| (C) Copyright National Semiconductor Corporation 2008
| and Teraspeed Consulting Group LLC 2008
|   National Semiconductor Corporation
|   Data Conversion Products Group
|   IBIS Model of ADC08D1000QML
|   128 Pin Quad Gullwing Ceramic Package
| Teraspeed Modeling Services.
| http://www.teraspeed.com
[IBIS Ver]  3.2
[File Name] adc08d1000qml.ibs
[File Rev]  3.3
[Source]  Created by Teraspeed Consulting Group LLC
[Date]   06/02/2008
[Notes]   Quality Check of this IBIS model: Model Passes IBIS Check
   Model parses into ICX IS. Simulation done with Hyperlynx.
   1. MIN TYP MAX information is based on Temprature and
   Voltage characteristics only.
   2. Package data gained using TDA Systems Iconnect Software.
[Disclaimer]
   All rights reserved
|   National Semiconductor Corporation hereby grants
|the user of this IBIS model a non-exclusive, nontransferable
|license to use this IBIS model under the following terms.
|Before using this IBIS model, the user should read this
|license.  If the user does not accept these terms,  the
|IBIS model should be returned to National within 30 days.
|   The user is granted this license only to use the
|IBIS model and is not granted rights to sell, load, rent,
|lease or license the IBIS model in whole or in part, or in
|modified form to anyone other than user. User may modify
|the IBIS model to suit its specific applications but rights
|to derivative works and such modifications shall belong to
|National.
|   This IBIS model is provided on an "AS IS" basis and
|National makes absolutely no warranty with respect to the
|information contained herein.NATIONAL DISCLAIMS AND CUSTOMER
|WAIVES ALL WARRANTIES, EXPRESS OR IMPLIED, INCLUDING
|WARRANTIES OF MERCHANTABILITY OR FITNESS FOR A PARTICULAR
|PURPOSE. The entire risk as to quality and performance is
|with the Customer. ACCORDINGLY, IN NO EVENT SHALL THE
|COMPANY BE LIABLE FOR ANY DAMAGES, WHETHER IN CONTRACT OR
|TORT,INCLUDING ANY LOST PROFITS OR OTHER INCIDENTAL,
|CONSEQUENTIAL, EXEMPLARY, OR PUNITIVE DAMAGES ARISING OUT
|OF THE USE OR APPLICATION OF THE IBIS model provided in
|this package.Further, National reserves the right to make
|changes without notice to any product herein to improve
|reliability, function, or design. National does not convey
|any license under patent rights or any other intellectual
|property rights, including those of third parties.
|   National is not obligated to provide maintenance or support
|for the licensed IBIS model.
| Use: Teraspeed Consulting Group LLC ("Teraspeed") has
| licensed IBIS models to specific integrated circuit
| suppliers ("IC Vendors") for use and distribution as
| follows: Each IC Vendor may use IBIS Models, and distribute
| them to IC Vendor's custumers to use solely for developing
| printed circute board designs. Users of this model may
| modify the IBIS model to suit its specific applications but
| rights to derivative works and such modifications shell belong
| to Teraspeed. No other distribution of these materials is
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[Copyright]
| This file is the legal property of National Semiconductor and
| Teraspeed Copyright(c) 2008.
| All other rights are reserved.
[Component]   ADC08D1000QML
[Manufacturer] National Semiconductor
[Package]
| variable   typ   min   max
R_pkg  1.000E-02  1.000E-02  1.000E-02
L_pkg  9.028E-09  8.236E-09  1.114E-08
C_pkg  2.390E-12  2.180E-12  2.950E-12
[Pin] signal_name  model_name  R_pin  L_pin C_pin
1   GND   GND   1.000E-02   1.114E-08   2.950E-12
2   VA   POWER   1.000E-02   1.081E-08   2.862E-12
3   OUTV/SCLK   in_ctrl   1.000E-02   1.050E-08   2.779E-12
4   OUTEDGE/DDR/SDATA   in_3lvl   1.000E-02   1.020E-08   2.700E-12
5   VA   POWER   1.000E-02   9.918E-09   2.625E-12
6   GND   GND   1.000E-02   9.653E-09   2.555E-12
7   VCMO   term   1.000E-02   9.408E-09   2.490E-12
8   VA   POWER   1.000E-02   9.183E-09   2.431E-12
9   GND   GND   1.000E-02   8.979E-09   2.377E-12
10   VINI-   term   1.000E-02   8.798E-09   2.329E-12
11   VINI+   term   1.000E-02   8.640E-09   2.287E-12
12   GND   GND   1.000E-02   8.507E-09   2.252E-12
13   VA   POWER   1.000E-02   8.399E-09   2.223E-12
14   FSR/ECE   in_rst   1.000E-02   8.318E-09   2.202E-12
15   DCLK_RST   in_rst   1.000E-02   8.263E-09   2.187E-12
16   VA   POWER   1.000E-02   8.236E-09   2.180E-12
17   VA   POWER   1.000E-02   8.236E-09   2.180E-12
18   CLK+   in_lvds   1.000E-02   6.040E-09   1.890E-12
19   CLK-   in_lvds   1.000E-02   5.750E-09   1.900E-12
20   VA   POWER   1.000E-02   8.399E-09   2.223E-12
21   GND   GND   1.000E-02   8.507E-09   2.252E-12
22   VINQ+   term   1.000E-02   8.640E-09   2.287E-12
23   VINQ-   term   1.000E-02   8.798E-09   2.329E-12
24   GND   GND   1.000E-02   8.979E-09   2.377E-12
25   VA   POWER   1.000E-02   9.183E-09   2.431E-12
26   PD   in_pd   1.000E-02   9.408E-09   2.490E-12
27   GND   GND   1.000E-02   9.653E-09   2.555E-12
28   VA   POWER   1.000E-02   9.918E-09   2.625E-12
29   PDQ   in_ctrl   1.000E-02   1.020E-08   2.700E-12
30   CAL   in_rst   1.000E-02   1.050E-08   2.779E-12
31   VBG   term   1.000E-02   1.081E-08   2.862E-12
32   REXT   term   1.000E-02   1.114E-08   2.950E-12
33   VA   POWER   1.000E-02   1.114E-08   2.950E-12
34   TDIODE_P   term   1.000E-02   1.081E-08   2.862E-12
35   TDIODE_N   term   1.000E-02   1.050E-08   2.779E-12
36   DQD0+   out_lvds  1.000E-02   1.020E-08   2.700E-12
37   DQD0-   out_lvds  1.000E-02   9.918E-09   2.625E-12
38   DQD1+   out_lvds  1.000E-02   9.653E-09   2.555E-12
39   DQD1-   out_lvds  1.000E-02   9.408E-09   2.490E-12
40   VDR   POWER   1.000E-02   9.183E-09   2.431E-12
41   _ECE   in_ctrl   1.000E-02   8.979E-09   2.377E-12
42   DRGND   GND   1.000E-02   8.798E-09   2.329E-12
43   DQD2+   out_lvds  1.000E-02   8.640E-09   2.287E-12
44   DQD2-   out_lvds  1.000E-02   8.507E-09   2.252E-12
45   DQD3+   out_lvds  1.000E-02   8.399E-09   2.223E-12
46   DQD3-   out_lvds  1.000E-02   8.318E-09   2.202E-12
47   DQD4+   out_lvds  1.000E-02   8.263E-09   2.187E-12
48   DQD4-   out_lvds  1.000E-02   8.236E-09   2.180E-12
49   DQD5+   out_lvds  1.000E-02   8.236E-09   2.180E-12
50   DQD5-   out_lvds  1.000E-02   8.263E-09   2.187E-12
51   VDR   POWER   1.000E-02   8.318E-09   2.202E-12
52   DRST_SEL   in_ctrl   1.000E-02   8.399E-09   2.223E-12
53   DRGND   GND   1.000E-02   8.507E-09   2.252E-12
54   DQD6+   out_lvds  1.000E-02   8.640E-09   2.287E-12
55   DQD6-   out_lvds  1.000E-02   8.798E-09   2.329E-12
56   DQD7+   out_lvds  1.000E-02   8.979E-09   2.377E-12
57   DQD7-   out_lvds  1.000E-02   9.183E-09   2.431E-12
58   DQ0+   out_lvds  1.000E-02   9.408E-09   2.490E-12
59   DQ0-   out_lvds  1.000E-02   9.653E-09   2.555E-12
60   DQ1+   out_lvds  1.000E-02   9.918E-09   2.625E-12
61   DQ1-   out_lvds  1.000E-02   1.020E-08   2.700E-12
62   VDR   POWER   1.000E-02   1.050E-08   2.779E-12
63   NC   NC   1.000E-02   1.081E-08   2.862E-12
64   DRGND   GND   1.000E-02   1.114E-08   2.950E-12
65   DQ2+   out_lvds  1.000E-02   1.114E-08   2.950E-12
66   DQ2-   out_lvds  1.000E-02   1.081E-08   2.862E-12
67   DQ3+   out_lvds  1.000E-02   1.050E-08   2.779E-12
68   DQ3-   out_lvds  1.000E-02   1.020E-08   2.700E-12
69   DQ4+   out_lvds  1.000E-02   9.918E-09   2.625E-12
70   DQ4-   out_lvds  1.000E-02   9.653E-09   2.555E-12
71   DQ5+   out_lvds  1.000E-02   9.408E-09   2.490E-12
72   DQ5-   out_lvds  1.000E-02   9.183E-09   2.431E-12
73   VDR   POWER   1.000E-02   8.979E-09   2.377E-12
74   DRGND   GND   1.000E-02   8.798E-09   2.329E-12
75   DQ6+   out_lvds  1.000E-02   8.640E-09   2.287E-12
76   DQ6-   out_lvds  1.000E-02   8.507E-09   2.252E-12
77   DQ7+   out_lvds  1.000E-02   8.399E-09   2.223E-12
78   DQ7-   out_lvds  1.000E-02   8.318E-09   2.202E-12
79   OR+/DCLK2+   out_lvds  1.000E-02   8.263E-09   2.187E-12
80   OR-/DCLK2-   out_lvds  1.000E-02   8.236E-09   2.180E-12
81   DCLK-   out_lvds  1.000E-02   8.236E-09   2.180E-12
82   DCLK+   out_lvds  1.000E-02   8.263E-09   2.187E-12
83   DI7-   out_lvds  1.000E-02   8.318E-09   2.202E-12
84   DI7+   out_lvds  1.000E-02   8.399E-09   2.223E-12
85   DI6-   out_lvds  1.000E-02   8.507E-09   2.252E-12
86   DI6+   out_lvds  1.000E-02   8.640E-09   2.287E-12
87   DRGND   GND   1.000E-02   8.798E-09   2.329E-12
88   VDR   POWER   1.000E-02   8.979E-09   2.377E-12
89   DI5-   out_lvds  1.000E-02   9.183E-09   2.431E-12
90   DI5+   out_lvds  1.000E-02   9.408E-09   2.490E-12
91   DI4-   out_lvds  1.000E-02   9.653E-09   2.555E-12
92   DI4+   out_lvds  1.000E-02   9.918E-09   2.625E-12
93   DI3-   out_lvds  1.000E-02   1.020E-08   2.700E-12
94   DI3+   out_lvds  1.000E-02   1.050E-08   2.779E-12
95   DI2-   out_lvds  1.000E-02   1.081E-08   2.862E-12
96   DI2+   out_lvds  1.000E-02   1.114E-08   2.950E-12
97   DRGND   GND   1.000E-02   1.114E-08   2.950E-12
98   NC   NC   1.000E-02   1.081E-08   2.862E-12
99   VDR   POWER   1.000E-02   1.050E-08   2.779E-12
100   DI1-   out_lvds  1.000E-02   1.020E-08   2.700E-12
101   DI1+   out_lvds  1.000E-02   9.918E-09   2.625E-12
102   DI0-   out_lvds  1.000E-02   9.653E-09   2.555E-12
103   DI0+   out_lvds  1.000E-02   9.408E-09   2.490E-12
104   DID7-   out_lvds  1.000E-02   9.183E-09   2.431E-12
105   DID7+   out_lvds  1.000E-02   8.979E-09   2.377E-12
106   DID6-   out_lvds  1.000E-02   8.798E-09   2.329E-12
107   DID6+   out_lvds  1.000E-02   8.640E-09   2.287E-12
108   DRGND   GND   1.000E-02   8.507E-09   2.252E-12
109   NC   NC   1.000E-02   8.399E-09   2.223E-12
110   VDR   POWER   1.000E-02   8.318E-09   2.202E-12
111   DID5-   out_lvds  1.000E-02   8.263E-09   2.187E-12
112   DID5+   out_lvds  1.000E-02   8.236E-09   2.180E-12
113   DID4-   out_lvds  1.000E-02   8.236E-09   2.180E-12
114   DID4+   out_lvds  1.000E-02   8.263E-09   2.187E-12
115   DID3-   out_lvds  1.000E-02   8.318E-09   2.202E-12
116   DID3+   out_lvds  1.000E-02   8.399E-09   2.223E-12
117   DID2-   out_lvds  1.000E-02   8.507E-09   2.252E-12
118   DID2+   out_lvds  1.000E-02   8.640E-09   2.287E-12
119   DRGND   GND   1.000E-02   8.798E-09   2.329E-12
120   NC   NC   1.000E-02   8.979E-09   2.377E-12
121   VDR   POWER   1.000E-02   9.183E-09   2.431E-12
122   DID1-   out_lvds  1.000E-02   9.408E-09   2.490E-12
123   DID1+   out_lvds  1.000E-02   9.653E-09   2.555E-12
124   DID0-   out_lvds  1.000E-02   9.918E-09   2.625E-12
125   DID0+   out_lvds  1.000E-02   1.020E-08   2.700E-12
126   CALRUN   out_cmos  1.000E-02   1.050E-08   2.779E-12
127   DES/_SCS   in_ctrl   1.000E-02   1.081E-08   2.862E-12
128   VA   POWER   1.000E-02   1.114E-08   2.950E-12
[Diff Pin] inv_pin vdiff tdelay_typ tdelay_min tdelay_max
11   10   NA   NA   NA   NA
18   19  200mV NA   NA   NA
22   23   NA   NA   NA   NA
36   37   NA   NA   NA   NA
38   39   NA   NA   NA   NA
43   44   NA   NA   NA   NA
45   46   NA   NA   NA   NA
47   48   NA   NA   NA   NA
49   50   NA   NA   NA   NA
54   55   NA   NA   NA   NA
56   57   NA   NA   NA   NA
58   59   NA   NA   NA   NA
60   61   NA   NA   NA   NA
65   66   NA   NA   NA   NA
67   68   NA   NA   NA   NA
69   70   NA   NA   NA   NA
71   72   NA   NA   NA   NA
75   76   NA   NA   NA   NA
77   78   NA   NA   NA   NA
79   80   NA   NA   NA   NA
82   81   NA   NA   NA   NA
84   83   NA   NA   NA   NA
86   85   NA   NA   NA   NA
90   89   NA   NA   NA   NA
92   91   NA   NA   NA   NA
94   93   NA   NA   NA   NA
96   95   NA   NA   NA   NA
101  100  NA   NA   NA   NA
103  102  NA   NA   NA   NA
105  104  NA   NA   NA   NA
107  106  NA   NA   NA   NA
112  111  NA   NA   NA   NA
114  113  NA   NA   NA   NA
116  115  NA   NA   NA   NA
118  117  NA   NA   NA   NA
123  122  NA   NA   NA   NA
125  124  NA   NA   NA   NA
[Series Pin Mapping] pin_2 model_name function_table_group
11   10   100_ohm
18   19   100_ohm
22   23   100_ohm
[Model Selector]  out_lvds
lvds_norm   normal amplitude lvds output
lvds_lo   reduced amplitude lvds output
[Model]   100_ohm
Model_type   Series
C_comp   0  0  0
[Temperature Range]   25   125   -55
|   typ   min   max
[Voltage Range]  1.9V 1.8V 2.0V
[R series]   100   94   106
[Model] term
Model_type Terminator
C_comp   0  0  0
| variable   typ   min   max
[Voltage Range]   1.900E+00   1.800E+00   2.000E+00
[POWER Clamp Reference]  1.900E+00   1.800E+00   2.000E+00
[GND Clamp Reference]   0.00000V   0.00000V   0.00000V
[Temperature Range]   25   125   -55
| Models and submodels in the file (10): in_3lvl (Input), in_ctrl (Input), in_lvds (Input), in_pd (Input), in_rst (Input), lvds_norm (Output), lvds_lo (Output), out_cmos (Output), 100_ohm (Series), term (Terminator)
